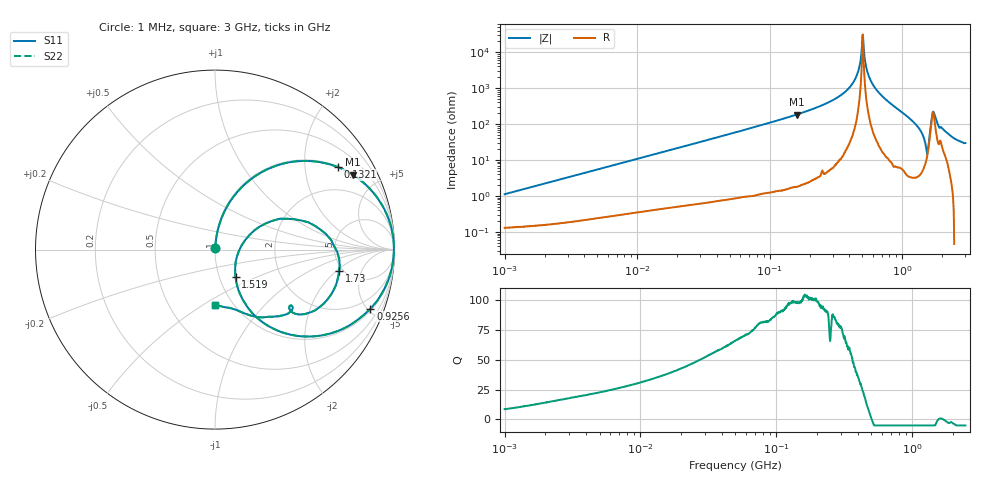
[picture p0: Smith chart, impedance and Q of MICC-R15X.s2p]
!s-Parameter Generated by FASTRON Sdn. Bhd.
!FASTRON P/N : MICC-R15X
!Keysight Technologies,E4991B,MY54100416,A.01.15
!Date: Wed Aug 26 15:50:46 2026
!Version  : Rev00 Wed Aug 26 15:50:46 2026
!Data & Calibration Information:
!PortZ  Port1:50+j0  Port2:50+j0
!When reading, reference impedance value at option line is always used.
!Remarks : This data is being provided solely for informational purposes.
!Freq	S11	S21	S12	S22
# Hz S dB R 50
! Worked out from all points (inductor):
!   1601 points, 1 MHz to 3 GHz, reference 50 ohm
!   read as one part in series: L = 176 nH near 1.041 MHz
!   highest Q = 102 at 159.8 MHz (marker M1), where L = 183 nH
!   self-resonance near 502.7 MHz
!   S11 on the Smith chart (normalised r, x): 1 MHz: 1.00, +0.02; 132.1 MHz: 1.03, +2.95; 925.6 MHz: 1.12, -5.22; 1.519 GHz: 1.19, -0.38; 1.73 GHz: 4.61, -2.20; 3 GHz: 0.82, -0.57
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1000000  -39.04 82.8  -0.01 -0.6  -0.01 -0.6  -39.04 82.8
3804036  -27.66 84.8  -0.03 -2.4  -0.03 -2.4  -27.66 84.8
1.447069e7  -16.37 79.7  -0.14 -8.7  -0.14 -8.7  -16.37 79.7
5.477226e7  -6.02 59.2  -1.32 -30.0  -1.32 -30.0  -6.02 59.2
1.321429e8  -1.69 34.0  -5.05 -55.4  -5.05 -55.4  -1.69 34.0
1.59818e8  -1.16 28.5  -6.44 -61.0  -6.44 -61.0  -1.16 28.5
2.083556e8  -0.64 21.2  -8.84 -68.2  -8.84 -68.2  -0.64 21.2
3.993203e8  -0.06 5.5  -20.30 -82.9  -20.30 -82.9  -0.06 5.5
4.548043e8  -0.03 2.5  -27.17 -83.9  -27.17 -83.9  -0.03 2.5
5.051982e8  -0.03 -0.0  -49.87 9.8  -49.87 9.8  -0.03 -0.0
5.473095e8  -0.04 -2.0  -28.92 82.1  -28.92 82.1  -0.04 -2.0
5.840965e8  -0.05 -3.8  -23.66 83.0  -23.66 83.0  -0.05 -3.8
7.925923e8  -0.30 -13.6  -12.55 74.9  -12.55 74.9  -0.30 -13.6
9.255909e8  -0.66 -20.8  -9.00 67.9  -9.00 67.9  -0.66 -20.8
1.313842e9  -4.05 -48.8  -2.46 38.8  -2.46 38.8  -4.05 -48.8
1.423359e9  -7.10 -58.5  -1.34 26.1  -1.34 26.1  -7.10 -58.5
1.519029e9  -14.39 -53.2  -0.93 9.8  -0.93 9.8  -14.39 -53.2
1.57318e9  -15.04 17.7  -1.59 -3.7  -1.59 -3.7  -15.04 17.7
1.629261e9  -7.18 23.1  -4.13 -16.0  -4.13 -16.0  -7.18 23.1
1.730092e9  -3.08 -10.0  -9.58 21.4  -9.58 21.4  -3.08 -10.0
1.874306e9  -4.61 -37.9  -3.80 34.0  -3.80 34.0  -4.61 -37.9
3e9  -10.16 -89.9  0.40 17.3  0.40 17.3  -10.16 -89.9
